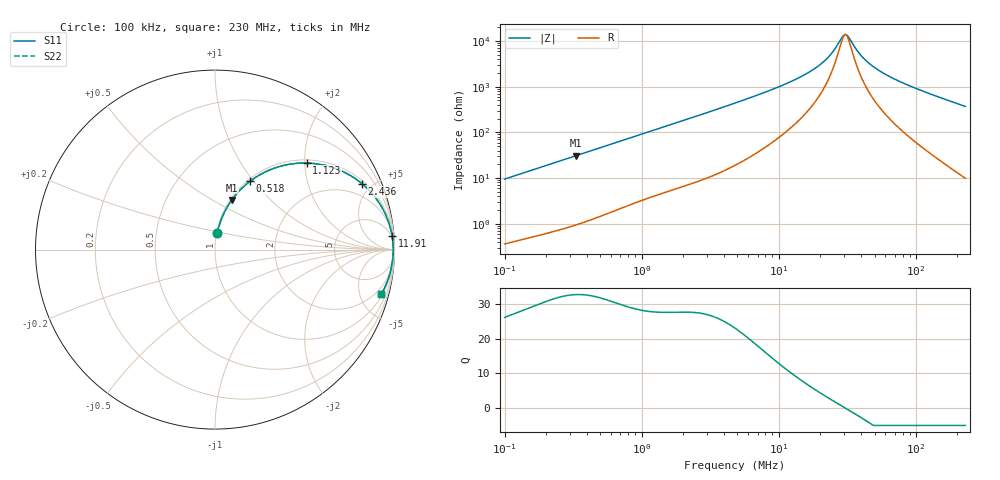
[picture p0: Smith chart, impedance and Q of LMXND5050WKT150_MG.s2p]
! LMXND5050WKT150_MG  S-PARAMETER MODEL  ( General Type )
! Model Generated by TAIYO YUDEN Corporation (https://www.yuden.co.jp/en/)
! Version 1.0
! TAIYO YUDEN Control No. 191023NI43SB-FBB
! Copyright(c) 2019 TAIYO YUDEN CO.,LTD. All Rights Reserved.
! Product Description (link to TY-COMPAS)
! https://ds.yuden.co.jp/TYCOMPAS/or/detail?pn=LMXND5050WKT150MMG&u=M
! Products Name : Inductors
! Characteristics :
!  Inductance : 15 uH , SRF(min) : 20 MHz , DC Resistance(max) : 0.198 Ohm
!  Rated Current : Saturation :1100 mA , Temp Rise : 1200 mA (40 degC)
!  Case Size : 4.9 x 4.9 / 0.193 x 0.193 [mm/inch] , Thickness : 2 / 0.079 [mm/inch]
!  (Conditions: Temperature = 25 degC , DC Bias Current/Voltage = 0A / 0V)
! External Node Assignments :
!  1  o---GGG---o  2
! GND o---------o GND
! Frequency Range : 0.1MHz  -  229.966873MHz  [ 402 STEP ]
# MHz S RI R 50
! Freq[MHz].  S11 Real  S11 Imag  S21 Real  S21 Imag  S12 Real  S12 Imag  S22 Real  S22 Imag
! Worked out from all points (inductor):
!   401 points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, 100 kHz to 230 MHz, reference 50 ohm
!   read as one part in series: L = 15 uH near 103.9 kHz
!   highest Q = 32.7 at 331.9 kHz (marker M1), where L = 14.8 uH
!   self-resonance near 30.15 MHz
!   S11 on the Smith chart (normalised r, x): 100 kHz: 1.01, +0.19; 518 kHz: 1.03, +0.96; 1.123 MHz: 1.07, +2.04; 2.436 MHz: 1.16, +4.39; 11.91 MHz: 3, +25; 230 MHz: 1.20, -7.37
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0.1  0.0124 0.0933  0.9876 -0.0933  0.9876 -0.0933  0.0124 0.0933
0.331939  0.0941 0.2771  0.9059 -0.2771  0.9059 -0.2771  0.0941 0.2771
0.365661  0.1108 0.299  0.8892 -0.299  0.8892 -0.299  0.1108 0.299
0.518029  0.1942 0.3801  0.8058 -0.3801  0.8058 -0.3801  0.1942 0.3801
0.792949  0.351 0.4605  0.649 -0.4605  0.649 -0.4605  0.351 0.4605
1.123364  0.511 0.4823  0.489 -0.4823  0.489 -0.4823  0.511 0.4823
1.337081  0.5922 0.4737  0.4078 -0.4737  0.4078 -0.4737  0.5922 0.4737
2.436054  0.8193 0.367  0.1807 -0.367  0.1807 -0.367  0.8193 0.367
4.889189  0.9439 0.2093  0.0561 -0.2093  0.0561 -0.2093  0.9439 0.2093
11.90771  0.9862 0.0786  0.0138 -0.0786  0.0138 -0.0786  0.9862 0.0786
17.53523  0.9909 0.0425  0.00912 -0.0425  0.00912 -0.0425  0.9909 0.0425
22.55099  0.9923 0.0225  0.00773 -0.0225  0.00773 -0.0225  0.9923 0.0225
25.3274  0.9926 0.0139  0.00739 -0.0139  0.00739 -0.0139  0.9926 0.0139
29.00146  0.9928 0.00397  0.00718 -0.00397  0.00718 -0.00397  0.9928 0.00397
30.73494  0.9928 -0.000236  0.00716 0.000236  0.00716 0.000236  0.9928 -0.000236
32.57203  0.9928 -0.00445  0.00717 0.00445  0.00717 0.00445  0.9928 -0.00445
38.02578  0.9926 -0.0158  0.00739 0.0158  0.00739 0.0158  0.9926 -0.0158
43.54189  0.9922 -0.026  0.00781 0.026  0.00781 0.026  0.9922 -0.026
51.82565  0.9913 -0.0398  0.00872 0.0398  0.00872 0.0398  0.9913 -0.0398
64.11956  0.9894 -0.0583  0.0106 0.0583  0.0106 0.0583  0.9894 -0.0583
110.2318  0.9785 -0.1186  0.0215 0.1186  0.0215 0.1186  0.9785 -0.1186
229.9669  0.9257 -0.2491  0.0743 0.2491  0.0743 0.2491  0.9257 -0.2491
